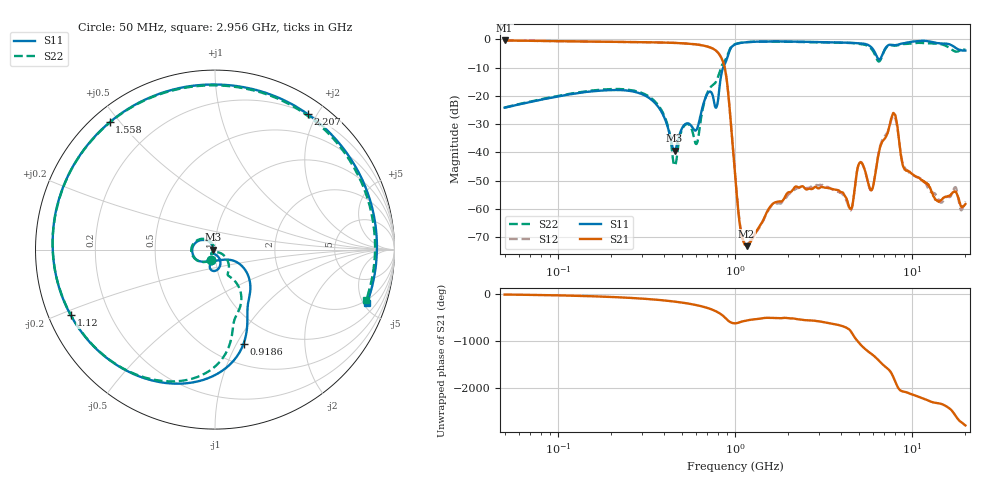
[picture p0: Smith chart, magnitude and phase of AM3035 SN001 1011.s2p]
# Hz S DB R 50
!freq MagS11 AngS11 MagS21 AngS21 MagS12 AngS12 MagS22 AngS22
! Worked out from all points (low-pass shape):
!   1601 points, 50 MHz to 20.05 GHz, reference 50 ohm
!   highest |S21| = -0.36 dB at 50 MHz (marker M1); lowest = -73.2 dB at 1.163 GHz (marker M2)
!   |S21| within 3 dB of the highest: start of sweep to 756.5 MHz
!   lowest |S11| = -39.3 dB at 455.9 MHz (marker M3), VSWR 1.02, Z = 48.9 - j0.0301 ohm
!   |S11| at or under -10 dB: start of sweep to 857.9 MHz
!   |S22| runs from -44.7 to -0.7 dB; largest |S21 - S12| = 0.0065
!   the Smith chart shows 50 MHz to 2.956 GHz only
!   S11 on the Smith chart (normalised r, x): 50 MHz: 0.95, -0.11; 918.6 MHz: 0.71, -1.07; 1.12 GHz: 0.06, -0.22; 1.558 GHz: 0.05, +0.47; 2.207 GHz: 0.20, +1.88; 2.956 GHz: 1.72, -5.31
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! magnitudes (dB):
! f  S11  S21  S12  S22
! 50 MHz  -24.2  -0.4  -0.4  -24.1
! 135.9 MHz  -18.8  -0.7  -0.7  -18.6
! 369.6 MHz  -23.9  -1.1  -1.1  -23.4
! 455.9 MHz  -39.3  -1.2  -1.2  -44.6
! 521.7 MHz  -30.1  -1.4  -1.4  -30.3
! 610.6 MHz  -31.7  -1.8  -1.8  -36.7
! 793.7 MHz  -23.3  -4.3  -4.3  -14.1
! 918.6 MHz  -5.2  -19.6  -19.7  -4.6
! 1.005 GHz  -1.7  -48.9  -48.5  -1.6
! 1.12 GHz  -1.1  -71.7  -71.5  -1.1
! 1.163 GHz  -1.0  -73.2  -72.5  -1.0
! 1.558 GHz  -0.7  -59.8  -60.1  -0.7
! 2.207 GHz  -0.8  -52.1  -52.9  -0.8
! 2.722 GHz  -0.9  -53.0  -52.3  -1.0
! 2.956 GHz  -0.9  -52.7  -51.6  -1.0
! 4.514 GHz  -1.2  -60.1  -60.5  -1.2
! 5.032 GHz  -1.4  -43.9  -43.8  -1.6
! 5.934 GHz  -2.9  -53.2  -53.3  -3.5
! 7.402 GHz  -2.0  -31.5  -31.7  -2.2
! 8.008 GHz  -2.0  -26.5  -27.5  -2.2
! 9.621 GHz  -1.0  -46.8  -47.1  -1.5
! 20.05 GHz  -3.9  -58.3  -57.3  -3.6
